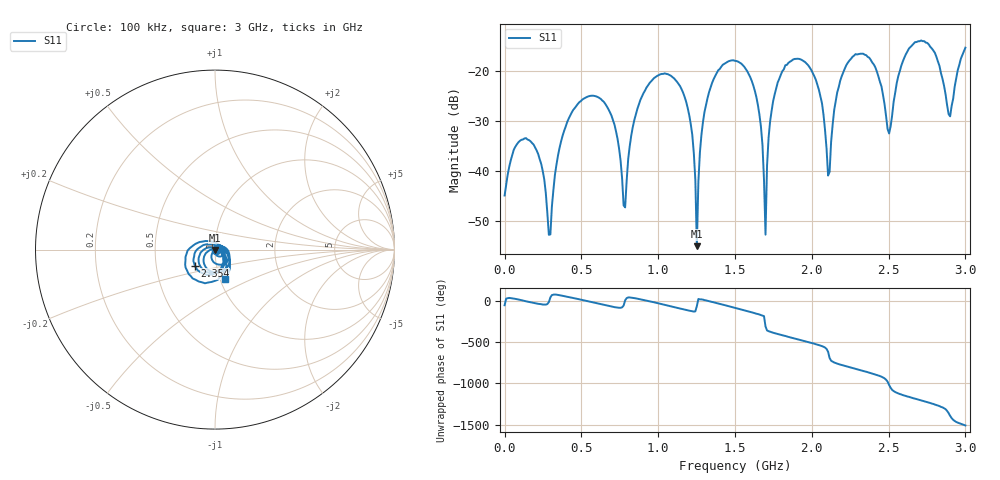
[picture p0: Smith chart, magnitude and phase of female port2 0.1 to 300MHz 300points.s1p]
# HZ S RI R 50
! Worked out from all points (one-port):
!   303 points, 100 kHz to 3 GHz, reference 50 ohm
!   lowest |S11| = -55.1 dB at 1.252 GHz (marker M1), VSWR 1.00, Z = 50.1 - j0.162 ohm
!   |S11| at or under -10 dB: start of sweep to end of sweep
!   S11 on the Smith chart (normalised r, x): 100 kHz: 1.01, -0.01; 2.354 GHz: 0.79, -0.15; 3 GHz: 1.06, -0.35
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100000  0.00314 -0.00473
1.689685e8  0.0187 -0.00678
2.981033e8  0.00181 0.00145
3.775708e8  0.012 0.0191
6.0604e8  0.0453 -0.0314
7.550417e8  0.000615 -0.0127
7.84842e8  0.00431 0.000221
8.841764e8  0.0496 0.0143
1.132513e9  -0.00205 -0.0745
1.221913e9  -0.0143 -0.018
1.251714e9  0.000715 -0.00161
1.271581e9  0.0149 0.00385
1.301381e9  0.0388 0.00376
1.50005e9  0.00425 -0.127
1.649052e9  -0.0438 -0.0136
1.678852e9  -0.0183 0.000601
1.698719e9  0.00158 0.00168
1.738453e9  0.0372 -0.0151
1.877521e9  -0.00728 -0.1306
2.036456e9  -0.0726 -0.00877
2.10599e9  -0.00173 0.00883
2.254992e9  -0.00308 -0.133
2.354326e9  -0.1125 -0.0909
2.503328e9  0.0122 0.0204
2.632462e9  0.016 -0.1681
2.801331e9  -0.1527 -0.00517
2.900665e9  0.0249 0.025
3e9  0.0565 -0.1627
